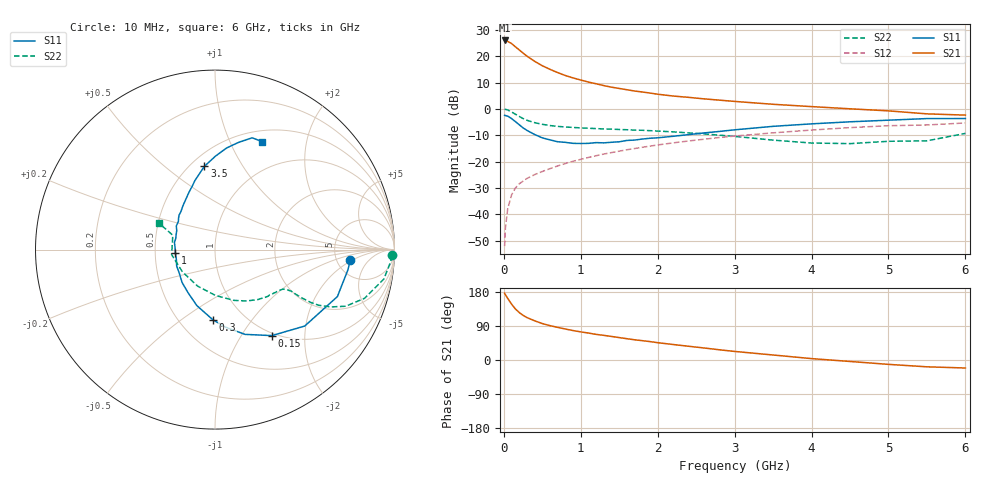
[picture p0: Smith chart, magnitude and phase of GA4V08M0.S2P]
! Infineon Technologies  Discrete & RF Semiconductors
! BF775
! Si NPN RF Bipolar Junction Transistor in SOT23
! VCE = 4 V  IC = 8 mA
! Common Emitter S-Parameters:  May  1996
# GHz  S  MA  R  50
!  f  S11  S21  S12  S22
! GHz  MAG  ANG  MAG  ANG  MAG  ANG  MAG  ANG
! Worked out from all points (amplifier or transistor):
!   36 points, 10 MHz to 6 GHz, reference 50 ohm
!   highest |S21| = 26.0 dB at 10 MHz (marker M1)
!   |S21| within 3 dB of that: start of sweep to 175.3 MHz
!   unconditionally stable (mu >= 1): 648.4 MHz to 3.141 GHz
!   at 250 MHz: K = 0.62, MSG = 24.3 dB, |S12| = -27.4 dB
!   at 1.4 GHz: K = 1.12, MAG = 10.3 dB, |S12| = -16.6 dB
!   at 6 GHz: K = 0.95, MSG = 1.5 dB, |S12| = -5.3 dB
!   S11 on the Smith chart (normalised r, x): 10 MHz: 6.65, -1.88; 150 MHz: 0.96, -1.38; 300 MHz: 0.72, -0.67; 1 GHz: 0.64, -0.03; 3.5 GHz: 0.58, +0.69; 6 GHz: 0.63, +1.33
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0.01  0.7559 -4.6  19.85 176.2  0.0025 88.9  0.9873 -1.9
0.02  0.749 -8.7  19.51 172.5  0.0055 86.5  0.9802 -4.1
0.05  0.7304 -21.0  19.07 162.6  0.0127 79.7  0.9549 -9.9
0.1  0.6569 -40.4  17.38 147.6  0.0233 72.0  0.8769 -18.0
0.15  0.5746 -56.5  15.04 134.8  0.0316 66.4  0.7942 -23.4
0.2  0.5011 -70.5  13.15 125.3  0.038 62.9  0.721 -26.3
0.25  0.4372 -82.0  11.44 117.8  0.0428 60.8  0.6567 -28.2
0.3  0.392 -91.6  10.02 112.0  0.048 60.9  0.6095 -28.9
0.4  0.3279 -108.0  7.994 103.5  0.0568 60.3  0.5493 -29.1
0.5  0.2826 -122.3  6.587 96.1  0.0651 61.4  0.5106 -28.9
0.6  0.259 -135.2  5.625 90.7  0.0737 61.9  0.4839 -28.6
0.7  0.2386 -146.4  4.881 86.1  0.0831 62.4  0.466 -29.0
0.8  0.2323 -156.8  4.296 81.7  0.0923 62.6  0.4545 -29.3
1  0.2214 -175.0  3.529 74.2  0.1106 62.8  0.4367 -30.3
1.1  0.2223 177.6  3.228 71.1  0.1202 62.6  0.4302 -31.5
1.3  0.2272 164.3  2.767 65.0  0.1395 61.9  0.4171 -33.8
1.6  0.2527 148.6  2.309 56.2  0.1682 60.1  0.4029 -38.1
2.2  0.3029 126.1  1.755 40.9  0.227 55.1  0.3675 -49.1
3.5  0.4675 97.3  1.224 13.2  0.352 40.4  0.256 -89.1
4.5  0.5697 83.5  1.005 -3.9  0.4419 27.5  0.2198 -145.5
5.5  0.6563 71.6  0.806 -18.0  0.4961 12.6  0.2483 161.2
6  0.657 66.3  0.763 -21.1  0.5417 8.6  0.3437 154.8
